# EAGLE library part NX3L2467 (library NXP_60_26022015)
The NX3L2467 is a dual low-ohmic double-pole double-throw analog switch suitable for use as an analog or digital multiplexer/demultiplexer. It consists of four switches, each with two independent input/outputs (nY0 and nY1) and a common input/output (nZ). The two digital inputs (1S and 2S) are used to select the switch position. 1S is used in selecting the independent inputs/outputs switched to 1Z and 2Z, and 2S is used in selecting the independent inputs/outputs switched to 3Z and 4Z. Schmitt trigger action at the select input (nS) makes the circuit tolerant to slower input rise and fall times across the entire VCC range from 1.4 V to 4.3 V. AAL Eindhoven MK
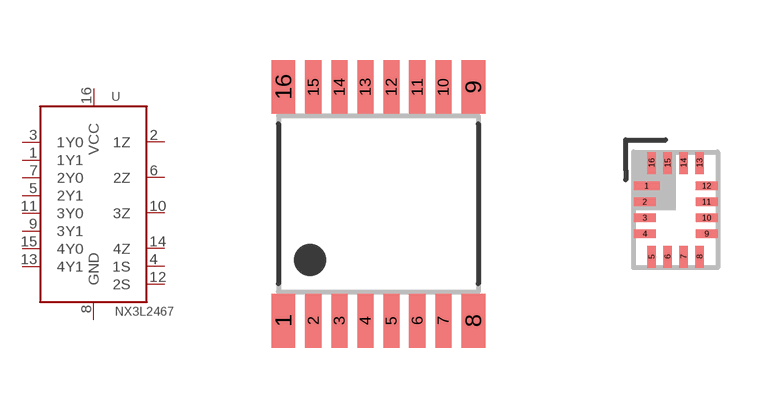
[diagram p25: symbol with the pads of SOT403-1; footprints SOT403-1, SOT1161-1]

Designator prefix U

## NX3L2467PW  [SOT403-1]
1  1Y1  in
2  1Z  out
3  1Y0  in
4  1S  in
5  2Y1  in
6  2Z  out
7  2Y0  in
8  GND  pwr
9  3Y1  in
10  3Z  out
11  3Y0  in
12  2S  in
13  4Y1  in
14  4Z  out
15  4Y0  in
16  VCC  pwr

## NX3L2467GU  [SOT1161-1]
1  1Y0  in
2  1S  in
3  2Y1  in
4  2Z  out
5  2Y0  in
6  GND  pwr
7  3Y1  in
8  3Z  out
9  3Y0  in
10  2S  in
11  4Y1  in
12  4Z  out
13  4Y0  in
14  VCC  pwr
15  1Y1  in
16  1Z  out

## NX3L2467HR  [SOT1039-2]
1  1Y0  in
2  1S  in
3  2Y1  in
4  2Z  out
5  2Y0  in
6  GND  pwr
7  3Y1  in
8  3Z  out
9  3Y0  in
10  2S  in
11  4Y1  in
12  4Z  out
13  4Y0  in
14  VCC  pwr
15  1Y1  in
16  1Z  out
CP  GND  pwr

## Footprint SOT403-1 (pad centres in mm)
SOT403-1 TSSOP16: plastic thin shrink small outline package; 16 leads; body width 4.4 mm JEDEC: MO-153 IEC: ---
smd 0.6 x 1.35: 1 -2.375,-2.925; 8 2.375,-2.925; 9 2.375,2.925; 16 -2.375,2.925
smd 0.4 x 1.35: 2 -1.625,-2.925; 3 -0.975,-2.925; 4 -0.325,-2.925; 5 0.325,-2.925; 6 0.975,-2.925; 7 1.625,-2.925; 10 1.625,2.925; 11 0.975,2.925; 12 0.325,2.925; 13 -0.325,2.925; 14 -0.975,2.925; 15 -1.625,2.925

## Footprint SOT1161-1 (pad centres in mm)
SOT1161-1 XQFN16: plastic, extremely thin quad flat package; no leads;16 terminals; body 1.80 x 2.60 x 0.50 mm JEDEC: -- IEC: --
smd 0.65 x 0.22: 1 -0.725,0.6
smd 0.55 x 0.22: 2 -0.775,0.2; 3 -0.775,-0.2; 4 -0.775,-0.6; 9 0.775,-0.6; 10 0.775,-0.2; 11 0.775,0.2; 12 0.775,0.6
smd 0.22 x 0.55: 5 -0.6,-1.175; 6 -0.2,-1.175; 7 0.2,-1.175; 8 0.6,-1.175; 13 0.6,1.175; 14 0.2,1.175; 15 -0.2,1.175; 16 -0.6,1.175

## Footprint SOT1039-2 (pad centres in mm)
SOT1039-2 HXQFN16: plastic thermal enhanced extremely thin quad flat package; no leads; 16 terminals; body 3 x 3 x 0.5 mm JEDEC: -- IEC: -- JEITA: --date: 2013-10-01
smd 0.85 x 0.24: 1 -1.575,0.75; 2 -1.575,0.25; 3 -1.575,-0.25; 4 -1.575,-0.75; 9 1.575,-0.75; 10 1.575,-0.25; 11 1.575,0.25; 12 1.575,0.75
smd 0.24 x 0.85: 5 -0.75,-1.575; 6 -0.25,-1.575; 7 0.25,-1.575; 8 0.75,-1.575; 13 0.75,1.575; 14 0.25,1.575; 15 -0.25,1.575; 16 -0.75,1.575
smd 1.8 x 1.8: CP 0,0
